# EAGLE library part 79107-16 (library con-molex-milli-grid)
RECEPTACAL
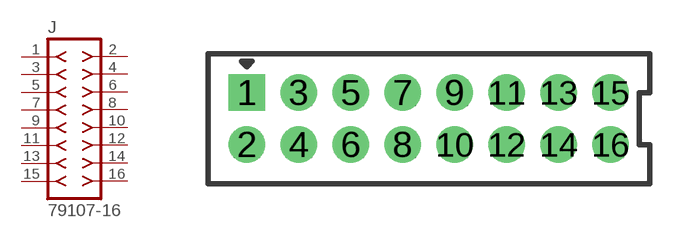
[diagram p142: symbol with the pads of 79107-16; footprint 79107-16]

Designator prefix J

## 79107-16  [79107-16]
1  1  pas
2  2  pas
3  3  pas
4  4  pas
5  5  pas
6  6  pas
7  7  pas
8  8  pas
9  9  pas
10  10  pas
11  11  pas
12  12  pas
13  13  pas
14  14  pas
15  15  pas
16  16  pas

## Footprint 79107-16 (pad centres in mm)
RECEPTACAL Dual Row, Vertical, Through-Hole
drill 0.914 square: 1 -7,1
drill 0.914: 2 -7,-1; 3 -5,1; 4 -5,-1; 5 -3,1; 6 -3,-1; 7 -1,1; 8 -1,-1; 9 1,1; 10 1,-1; 11 3,1; 12 3,-1; 13 5,1; 14 5,-1; 15 7,1; 16 7,-1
